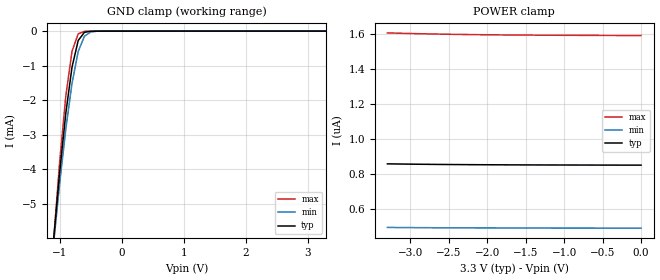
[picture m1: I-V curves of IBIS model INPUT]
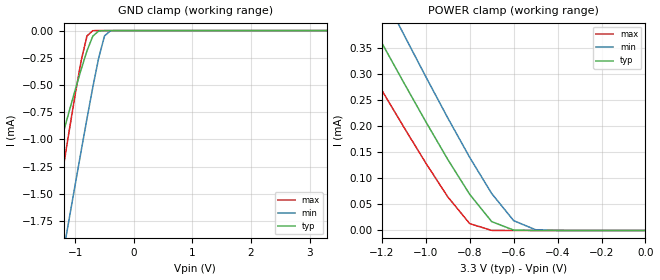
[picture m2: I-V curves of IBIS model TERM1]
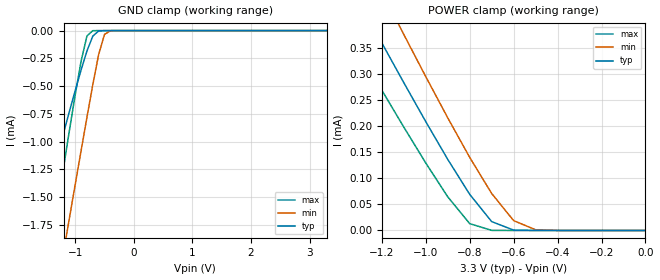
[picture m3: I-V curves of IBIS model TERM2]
|   PERICOM SEMICONDUCTOR CORP
|   IBIS Model of PI3L500-a
|   Product Family: 3L
|   TQFN (ZF-56PIN) Package
[IBIS Ver] 3.2
[Comment char] |_char
[File Name] pi3l500-a_zf_reva.ibs
[File Rev] 1.1
[Source] File originated at Pericom Semiconductor Corp.
[Date] 10/27/17
[Disclaimer] (C) Copyright PERICOM Semiconductor Corporation
   All rights reserved
  Pericom Semiconductor Corporation hereby grants the user of
  this IBIS model a non-exclusive, nontransferable license to
  use this IBIS model under the following terms.
  This IBIS model is provided on an "AS IS" basis and Pericom
  makes absolutely no warranty with respect to the information
  contained herein. PERICOM DISCLAIMS AND CUSTOMER WAIVES ALL
  WARRANTIES, EXPRESSED OR IMPLIED, INCLUDING WARRANTIES OF
  MERCHANTABILITY OR FITNESS FOR A PARTICULAR PURPOSE. The
  entire risk as to quality and performance is with the customer.
  Accordingly, in no event shall the company be liable for any
  damages, whether in contract or tort, including any lost
  profits or other incidental, consequential, exemplary, or
  punitive damages arising out of the use or application of the
  IBIS model provided in this package. Further, Pericom reserves
  the right to make changes without notice to any product herein
  to improve reliability, function, or design. Pericom does not
  convey any license under patent rights or any other intellectual
  property rights, including those of third parties.
  The user is granted this license only to use the IBIS model
  and is not granted rights to sell, load, rent, lease or license
  the IBIS model in whole or in part, or in modified form to anyone
  other than user. User may modify the IBIS model to suit its specific
  application but rights to derivative works and such modifications
  shall belong to Pericom.
  Pericom is not obligated to provide maintenance or support
  for the licensed IBIS model.
  Contact Pericom at ATTN: APPLICATION ENGINEERING / IBIS MODELS
  1545 Barber Lane Milpitas, CA 95035 USA.
[Component] PI3L500-A
[Manufacturer] Pericom Semiconductor Corp.
[Package]
| variable   typ   min   max
R_pkg   0.07037ohm   0.04680ohm   0.09394ohm
L_pkg   2.25802nH   1.50075nH   3.01529nH
C_pkg   0.09446pF   0.03924pF   0.14969pF
[Pin] signal_name   model_name   R_pin   L_pin   C_pin
1   GND   GND   0.08662   2.77957nH   0.12989pF
2   A0   TERM1   0.08855   2.84005nH   0.10569pF
3   A1   TERM1   0.08265   2.65099nH   0.09541pF
4   VCC   POWER   0.07370   2.36462nH   0.08990pF
5   NC   NC   0.06646   2.19710nH   0.07511pF
6   GND   GND   0.05935   1.90318nH   0.05906pF
7   A2   TERM1   0.05868   1.88121nH   0.05546pF
8   A3   TERM1   0.05586   1.79102nH   0.05566pF
9   GND   GND   0.04908   1.57337nH   0.04266pF
10   VCC   POWER   0.04731   1.51498nH   0.03924pF
11   A4   TERM1   0.05046   1.61763nH   0.04587pF
12   A5   TERM1   0.05094   1.63312nH   0.04716pF
13   GND   GND   0.04883   1.56563nH   0.04354pF
14   A6   TERM1   0.05467   1.75284nH   0.05297pF
15   A7   TERM1   0.05800   1.85909nH   0.05364pF
16   GND   GND   0.05788   1.85468nH   0.04949pF
17   SEL   INPUT   0.06308   2.02131nH   0.05883pF
18   VCC   POWER   0.06882   2.20570nH   0.06921pF
19   LED0   TERM1   0.07434   2.38146nH   0.08257pF
20   LED1   TERM1   0.08040   2.57965nH   0.12182pF
21   GND   GND   0.08186   2.62579nH   0.11928pF
22   0LED1   TERM2   0.07809   2.50287nH   0.08095pF
23   1LED1   TERM2   0.07532   2.41352nH   0.07014pF
24   GND   GND   0.07358   2.35774nH   0.06537pF
25   0LED2   TERM2   0.07343   2.35294nH   0.06474pF
26   1LED2   TERM2   0.07439   2.38366nH   0.06792pF
27   VCC   POWER   0.07668   2.45807nH   0.08086pF
28   GND   GND   0.09182   2.94599nH   0.14764pF
29   7B2   TERM2   0.09394   3.01529nH   0.14969pF
30   6B2   TERM2   0.08878   2.84841nH   0.11000pF
31   7B1   TERM2   0.08316   2.66761nH   0.09542pF
32   6B1   TERM2   0.07703   2.47085nH   0.08494pF
33   GND   GND   0.07082   2.27153nH   0.07619pF
34   5B2   TERM2   0.06502   2.08547nH   0.06858pF
35   4B2   TERM2   0.05901   1.89246nH   0.06012pF
36   5B1   TERM2   0.05379   1.72506nH   0.05309pF
37   4B1   TERM2   0.04981   1.59730nH   0.04720pF
38   VCC   POWER   0.04727   1.51568nH   0.04279pF
39   GND   GND   0.04680   1.50075nH   0.04210pF
40   3B2   TERM2   0.04847   1.55444nH   0.04519pF
41   2B2   TERM2   0.05177   1.66038nH   0.05042pF
42   3B1   TERM2   0.05646   1.81066nH   0.05700pF
43   2B1   TERM2   0.06208   1.99103nH   0.06512pF
44   GND   GND   0.06761   2.16871nH   0.07252pF
45   1B2   TERM2   0.07362   2.36152nH   0.08107pF
46   0B2   TERM2   0.07960   2.55347nH   0.09129pF
47   1B1   TERM2   0.08511   2.73082nH   0.10544pF
48   0B1   TERM2   0.09020   2.89509nH   0.14372pF
49   GND   GND   0.08781   2.81752nH   0.13842pF
50   VCC   POWER   0.07697   2.46803nH   0.08357pF
51   2LED1   TERM2   0.07467   2.39354nH   0.07187pF
52   2LED2   TERM2   0.07345   2.35412nH   0.06765pF
53   GND   GND   0.07337   2.35183nH   0.06788pF
54   LED2   TERM1   0.07458   2.39069nH   0.07201pF
55   GND   GND   0.07691   2.46576nH   0.08252pF
56   VCC   POWER   0.08557   2.74545nH   0.13180pF
[Series Switch Groups]
On 1 /
Off 2 /
[Series_Pin_Mapping]   pin_2   model_name   function_table_group
2   48   SWITCH1   1
3   47   SWITCH1   1
7   43   SWITCH1   1
8   42   SWITCH1   1
11   37   SWITCH1   1
12   36   SWITCH1   1
14   32   SWITCH1   1
15   31   SWITCH1   1
19   22   SWITCH1   1
20   23   SWITCH1   1
54   52   SWITCH1   1
2   46   SWITCH1   2
3   45   SWITCH1   2
7   41   SWITCH1   2
8   40   SWITCH1   2
11   35   SWITCH1   2
12   34   SWITCH1   2
14   30   SWITCH1   2
15   29   SWITCH1   2
19   25   SWITCH1   2
20   26   SWITCH1   2
54   51   SWITCH1   2
|   Model SWITCH1
[Model] SWITCH1
Model_type Series_switch
| variable   typ   min   max
C_comp   8.0000pF   7.9200pF   8.0800pF
[Voltage Range]   3.3000V   3.0000V   3.6000V
[temperature range]   25   85   -40
[On]
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[OFF]
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| Models and submodels in the file (4): INPUT (Input), SWITCH1 (Series_switch), TERM1 (Terminator), TERM2 (Terminator)
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|   Model INPUT
[Model] INPUT
Model_type Input
Vinl = 0.800V
Vinh = 2.000V
| variable   typ   min   max
C_comp   6.0000pF   5.9400pF   6.0600pF
[Voltage Range]   3.3000V   3.0000V   3.6000V
[temperature range]   25   85   -40
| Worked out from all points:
|   GND clamp passes 1 mA (typ) near -0.79 V on its own axis
[GND Clamp]
| Voltage   I(typ)   I(min)   I(max)
-3.3V     -68.99mA   -61.28mA   -79.71mA
-1.1V     -6.106mA   -6.219mA   -6.143mA
-1V       -4.105mA   -4.429mA   -3.806mA
-900mV    -2.379mA   -2.835mA   -1.883mA
-800mV    -1.044mA   -1.512mA   -584.2uA
-700mV    -271.4uA   -589uA     -77.64uA
-600mV    -35.44uA   -150uA     -5.462uA
-500mV    -3.314uA   -24.02uA   -1.072uA
-400mV    -593.3nA   -2.13uA    -741.6nA
3.3V      848.5nA    488.8nA    1.588uA
[POWER Clamp]
| Voltage   I(typ)   I(min)   I(max)
-3.3V     856nA      492.7nA    1.604uA
-3.1V     854.8nA    492.1nA    1.602uA
-3V       854.3nA    491.8nA    1.6uA
-2.9V     853.8nA    491.6nA    1.599uA
-2.7V     852.9nA    491.1nA    1.598uA
-2.4V     851.8nA    490.5nA    1.595uA
-2.2V     851.3nA    490.2nA    1.594uA
-2V       850.8nA    490nA      1.593uA
-1.6V     850.1nA    489.6nA    1.592uA
-1.2V     849.6nA    489.3nA    1.591uA
-800mV    849.2nA    489.1nA    1.59uA
0V        848.5nA    488.6nA    1.589uA
|   Model TERM1
[Model] TERM1
Model_type Terminator
| variable   typ   min   max
C_comp   4.0000pF   3.9600pF   4.0400pF
[Voltage Range]   3.3000V   3.0000V   3.6000V
[temperature range]   25   85   -40
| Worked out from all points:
|   GND clamp passes 1 mA (typ) near -1.24 V on its own axis
|   POWER clamp passes 1 mA (typ) near -2.02 V on its own axis
[GND Clamp]
| Voltage   I(typ)   I(min)   I(max)
-3.3V     -5.189mA   -8.606mA   -8.624mA
-1.7V     -1.926mA   -3.581mA   -2.972mA
-1.6V     -1.725mA   -3.269mA   -2.623mA
-1.4V     -1.325mA   -2.646mA   -1.929mA
-1.2V     -929.2uA   -2.027mA   -1.245mA
-1.1V     -734.6uA   -1.719mA   -909.8uA
-900mV    -358.6uA   -1.109mA   -280.1uA
-800mV    -186.6uA   -809.8uA   -49.22uA
-700mV    -50.86uA   -519.5uA   -680.8nA
-500mV    -378.7nA   -48.65uA   -222.7pA
-400mV    -8.083nA   -2.148uA   -84.11pA
3.3V      193.3pA    2.231nA    191.2pA
[POWER Clamp]
| Voltage   I(typ)   I(min)   I(max)
-3.3V     2.022mA    2.245mA    1.816mA
-1.4V     513.2uA    622.9uA    412uA
-1.3V     435.7uA    539.6uA    339.8uA
-1.2V     358.8uA    456.9uA    268.3uA
-1.1V     282.8uA    375uA      197.8uA
-1V       208.2uA    294.3uA    129.1uA
-900mV    136uA      215.4uA    64.36uA
-800mV    69.05uA    139.8uA    13.06uA
-700mV    16.97uA    70.73uA    200.9nA
-600mV    728.1nA    18.8uA     1.569nA
-500mV    14.88nA    1.363uA    252.3pA
0V        193.3pA    179.7pA    210.9pA
|   Model TERM2
[Model] TERM2
Model_type Terminator
| variable   typ   min   max
C_comp   4.0000pF   3.9600pF   4.0400pF
[Voltage Range]   3.3000V   3.0000V   3.6000V
[temperature range]   25   85   -40
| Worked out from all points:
|   GND clamp passes 1 mA (typ) near -1.24 V on its own axis
|   POWER clamp passes 1 mA (typ) near -2.02 V on its own axis
[GND Clamp]
| Voltage   I(typ)   I(min)   I(max)
-3.3V     -5.176mA   -8.558mA   -8.595mA
-1.7V     -1.919mA   -3.549mA   -2.957mA
-1.6V     -1.718mA   -3.237mA   -2.609mA
-1.4V     -1.318mA   -2.616mA   -1.917mA
-1.3V     -1.12mA    -2.307mA   -1.574mA
-1.1V     -729.5uA   -1.691mA   -901uA
-900mV    -354.8uA   -1.082mA   -275.6uA
-800mV    -183.7uA   -781.3uA   -48.4uA
-700mV    -49.69uA   -487uA     -679.6nA
-500mV    -368.7nA   -34.56uA   -222.6pA
-400mV    -7.999nA   -1.772uA   -84.1pA
3.3V      112.8pA    2.148nA    111.3pA
[POWER Clamp]
| Voltage   I(typ)   I(min)   I(max)
-3.3V     2.022mA    2.245mA    1.816mA
-1.4V     513.2uA    622.9uA    412uA
-1.3V     435.7uA    539.6uA    339.8uA
-1.2V     358.8uA    456.9uA    268.3uA
-1.1V     282.8uA    375uA      197.8uA
-1V       208.2uA    294.3uA    129.1uA
-900mV    136uA      215.4uA    64.36uA
-800mV    69.05uA    139.8uA    13.06uA
-700mV    16.97uA    70.73uA    200.8nA
-600mV    728nA      18.8uA     1.465nA
-500mV    14.79nA    1.363uA    151.4pA
0V        112.8pA    104.9pA    123.1pA
